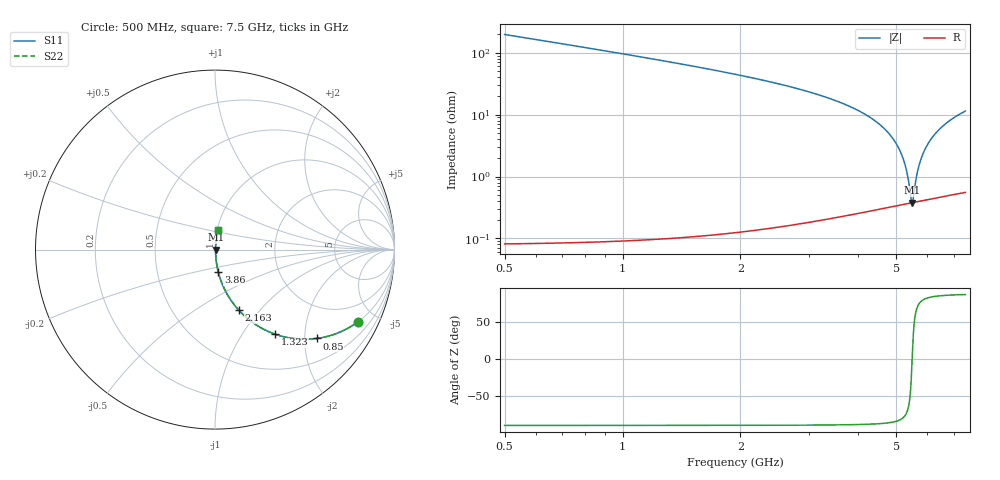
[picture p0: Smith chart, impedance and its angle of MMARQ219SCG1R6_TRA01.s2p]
! MMARQ219SCG1R6_TRA01  S-PARAMETER MODEL  ( General Type )
! Model Generated by TAIYO YUDEN Corporation (http://www.ty-top.com)
! Version 1.0
! TAIYO YUDEN Control No. 180601
! Copyright(c) 2018 TAIYO YUDEN CO.,LTD. All Rights Reserved.
! Product Description (link to TY-COMPAS)
! https://ds.yuden.co.jp/TYCOMPAS/or/detail?pn=MMARQ219SCG1R6BTRA01&u=M
! Products Name : Multilayer Ceramic Capacitors
! Characteristics :
!  Capacitance : 1.6 pF , Rated Voltage : 250V , TCC : CG / C0G
!  Case Size : 2.0 x 1.25 / 0.079 x 0.049 [mm/inch] , Thickness : 0.85 / 0.033 [mm/inch]
!  (Conditions: Temperature = 25 degC , DC Bias Current/Voltage = 0A / 0V)
! External Node Assignments :
!  1  o---| |---o  2
! GND o---------o GND
! Frequency Range : 500MHz  -  7500MHz  [ 401 STEP ]
# MHz S RI R 50
! Freq[MHz].  S11 Real  S11 Imag  S21 Real  S21 Imag  S12 Real  S12 Imag  S22 Real  S22 Imag
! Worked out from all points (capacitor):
!   401 points, 500 MHz to 7.5 GHz, reference 50 ohm
!   read as one part in series: C = 1.6 pF near 535 MHz
!   lowest |Z| = 377 mohm at 5.487 GHz (marker M1)
!   series resonance near 5.485 GHz, so ESL is about 530 pH
!   S11 on the Smith chart (normalised r, x): 500 MHz: 1.00, -3.95; 850 MHz: 1.00, -2.28; 1.323 GHz: 1.00, -1.42; 2.163 GHz: 1.00, -0.78; 3.86 GHz: 1.00, -0.26; 7.5 GHz: 1.01, +0.23
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500  0.7956 -0.4031  0.2044 0.4031  0.2044 0.4031  0.7956 -0.4031
850  0.5661 -0.4952  0.4339 0.4952  0.4339 0.4952  0.5661 -0.4952
1322.5  0.3343 -0.4711  0.6657 0.4711  0.6657 0.4711  0.3343 -0.4711
1672.5  0.2258 -0.417  0.7742 0.417  0.7742 0.417  0.2258 -0.417
2162.5  0.1318 -0.3365  0.8682 0.3365  0.8682 0.3365  0.1318 -0.3365
2845  0.0625 -0.2388  0.9375 0.2388  0.9375 0.2388  0.0625 -0.2388
3860  0.0188 -0.1269  0.9812 0.1269  0.9812 0.1269  0.0188 -0.1269
4000  0.0157 -0.1139  0.9843 0.1139  0.9843 0.1139  0.0157 -0.1139
4402.5  0.00916 -0.0791  0.9908 0.0791  0.9908 0.0791  0.00916 -0.0791
4735  0.00592 -0.0528  0.9941 0.0528  0.9941 0.0528  0.00592 -0.0528
4980  0.00453 -0.0346  0.9955 0.0346  0.9955 0.0346  0.00453 -0.0346
5172.5  0.00393 -0.021  0.9961 0.021  0.9961 0.021  0.00393 -0.021
5312.5  0.00374 -0.0115  0.9963 0.0115  0.9963 0.0115  0.00374 -0.0115
5452.5  0.00373 -0.00214  0.9963 0.00214  0.9963 0.00214  0.00373 -0.00214
5487.5  0.00376 0.000152  0.9962 -0.000152  0.9962 -0.000152  0.00376 0.000152
5522.5  0.00379 0.00243  0.9962 -0.00243  0.9962 -0.00243  0.00379 0.00243
5662.5  0.00404 0.0114  0.996 -0.0114  0.996 -0.0114  0.00404 0.0114
5802.5  0.00444 0.0201  0.9956 -0.0201  0.9956 -0.0201  0.00444 0.0201
6030  0.00538 0.0338  0.9946 -0.0338  0.9946 -0.0338  0.00538 0.0338
6345  0.00723 0.052  0.9928 -0.052  0.9928 -0.052  0.00723 0.052
6852.5  0.0113 0.0794  0.9887 -0.0794  0.9887 -0.0794  0.0113 0.0794
7500  0.0182 0.1115  0.9818 -0.1115  0.9818 -0.1115  0.0182 0.1115
